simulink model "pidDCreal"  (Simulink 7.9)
settings: Solver=ode1  SolverMode=SingleTasking  StartTime=0.0  StopTime=49  FixedStep=Ts  RelTol=1e-3  AbsTol=1e-6
PreLoadFcn:
  | pidDCinit
InitFcn:
  | pidDCinit
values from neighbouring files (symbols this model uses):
  Ts = 0.1    [pidDCinit.m]    (also in stupidDCinit.m; da_bode_evolution.m = 1)
undefined symbols (not defined in the file or in its folder): DiscIntNeverNeededParam

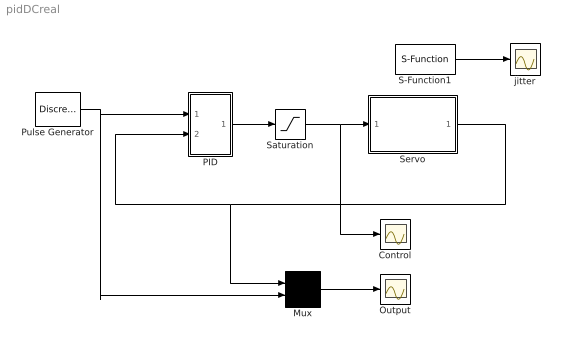
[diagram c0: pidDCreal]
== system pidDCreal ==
  Control : Scope
  Mux : Mux  Inputs=2
  Output : Scope
  PID : Subsystem  mask{K=1.7, Ti=1.15, Td=0.3}
      mask init:
      | b_reg=1; c_reg=0;
  Pulse Generator : DiscretePulseGenerator  PulseType=Time based  Amplitude=2  Period=10  PulseWidth=50
  S-Function1 : S-Function  FunctionName=realtimer  Parameters=Ts  EnableBusSupport=off
  Saturation : Saturate  UpperLimit=10  LowerLimit=-10
  Servo : Subsystem
  jitter : Scope
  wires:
  Mux/1 -> Output/1
  Pulse Generator/1 -> Mux/2, PID/1(uc)
  PID/1(Out1) -> Saturation/1
  Servo/1(p_2) -> Mux/1, PID/2(y)
  S-Function1/1 -> jitter/1
  Saturation/1 -> Servo/1(u), Control/1

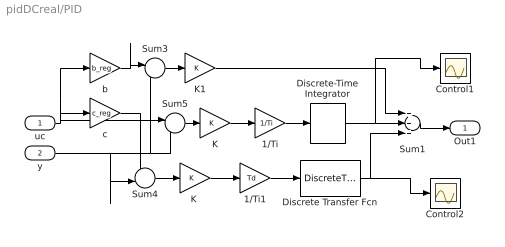
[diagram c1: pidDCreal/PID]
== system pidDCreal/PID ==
  uc : Inport
  y : Inport  Port=2
  1/Ti : Gain  Gain=1/Ti
  1/Ti1 : Gain  Gain=Td
  Control1 : Scope
  Control2 : Scope
  Discrete Transfer Fcn : DiscreteTransferFcn  Numerator=[1 -1]*1/(Td/10+Ts)  Denominator=[1 -Td/(Td+10*Ts)]  SampleTime=Ts
  Discrete-Time Integrator : DiscreteIntegrator  SampleTime=Ts  ICPrevOutput=DiscIntNeverNeededParam  ICPrevScaledInput=DiscIntNeverNeededParam
  K : Gain  Gain=K
  "K " : Gain  Gain=K
  K1 : Gain  Gain=K
  Sum1 : Sum  Inputs=+++
  Sum3 : Sum  Inputs=+-
  Sum4 : Sum  Inputs=+-
  Sum5 : Sum  Inputs=+-
  b : Gain  Gain=b_reg
  c : Gain  Gain=c_reg
  Out1 : Outport
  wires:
  K/1 -> 1/Ti/1
  1/Ti/1 -> Discrete-Time Integrator/1
  Sum1/1 -> Out1/1
  Discrete-Time Integrator/1 -> Sum1/2, Control1/1
  Discrete Transfer Fcn/1 -> Sum1/3, Control2/1
  1/Ti1/1 -> Discrete Transfer Fcn/1
  "K "/1 -> 1/Ti1/1
  uc/1 -> c/1, b/1, Sum5/1
  b/1 -> Sum3/1
  y/1 -> Sum4/2, Sum3/2, Sum5/2
  Sum3/1 -> K1/1
  K1/1 -> Sum1/1
  c/1 -> Sum4/1
  Sum4/1 -> "K "/1
  Sum5/1 -> K/1

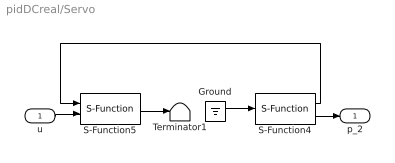
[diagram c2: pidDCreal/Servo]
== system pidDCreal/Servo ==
  u : Inport
  Ground : Ground
  S-Function4 : S-Function  FunctionName=analogin  Parameters=Ts [0]  EnableBusSupport=off
  S-Function5 : S-Function  FunctionName=analogout  Parameters=Ts [0]  EnableBusSupport=off
  Terminator1 : Terminator
  p_2 : Outport
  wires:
  Ground/1 -> S-Function4/1
  S-Function5/1 -> Terminator1/1
  S-Function4/1 -> S-Function5/1
  S-Function4/2 -> p_2/1
  u/1 -> S-Function5/2
